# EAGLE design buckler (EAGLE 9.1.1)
AUTHOR: Branden Ghena; REV: B; TITLE: Berkeley Buckler

## Sheet 1 of 3: Headers
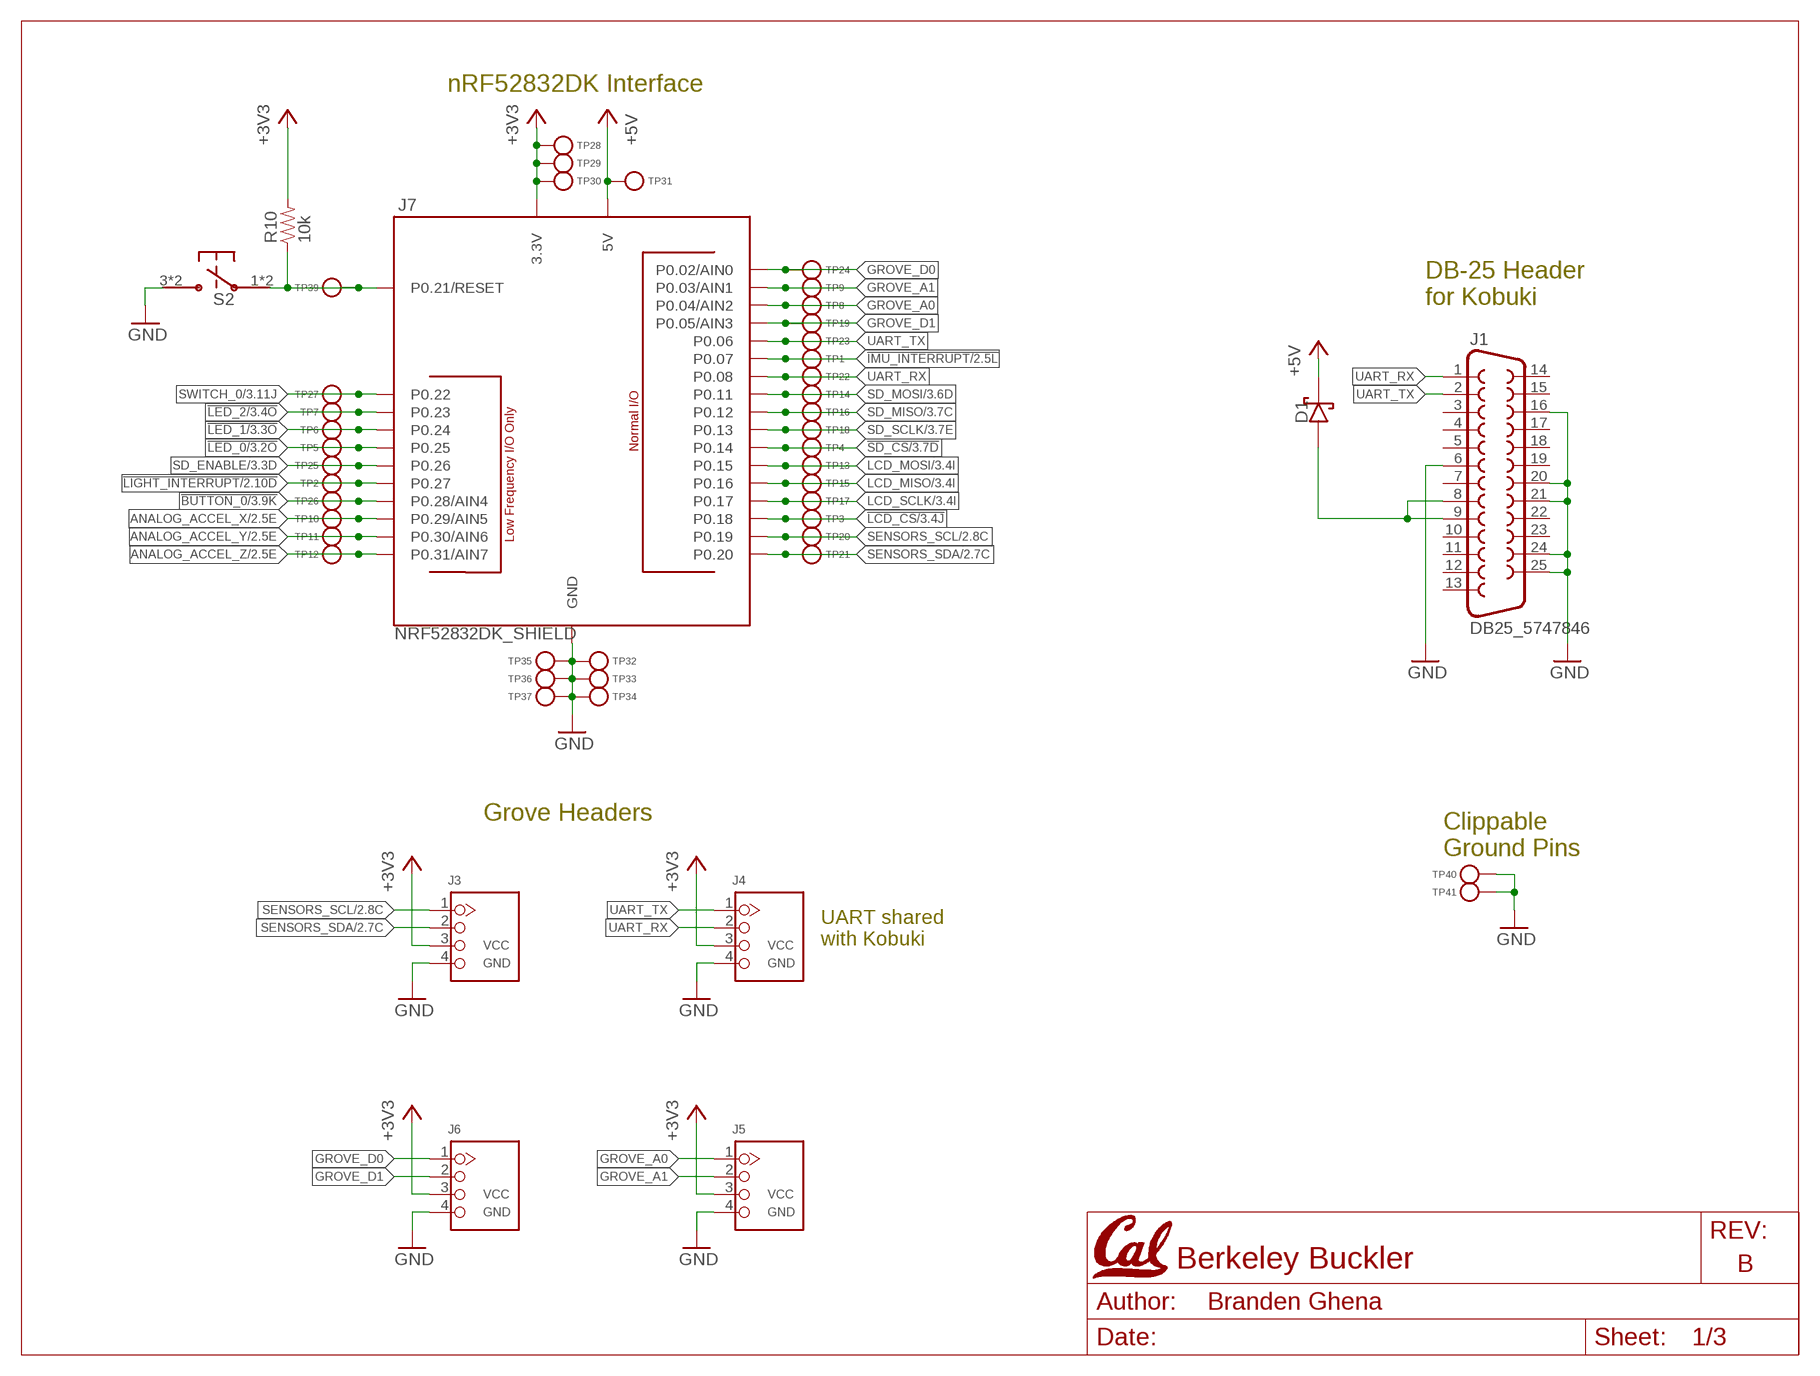
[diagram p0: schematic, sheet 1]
U$1 (LETTER_L_CAL): HEIGHT: 8.5in; WIDTH: 11in

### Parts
D1  DIODE_SCHOTTKYSOD323  [SOD323]
J1  DB25_5747846  [DB25_5747846]
J3  GROVE-CONNECTOR-DIP(4P-2.0)  [HW4-2.0]
J4  GROVE-CONNECTOR-DIP(4P-2.0)  [HW4-2.0]
J5  GROVE-CONNECTOR-DIP(4P-2.0)  [HW4-2.0]
J6  GROVE-CONNECTOR-DIP(4P-2.0)  [HW4-2.0]
J7  NRF52832DK_SHIELD  [NRF52832DK_SHIELD]
R10  10k  RESISTOR0402_RES  [0402_RES]
S2  PTS645SM43SMTR92  [PTS645]
TP1  TEST_POINT_0.040IN  [TESTPOINT_0.040IN]
TP2  TEST_POINT_0.040IN  [TESTPOINT_0.040IN]
TP3  TEST_POINT_0.040IN  [TESTPOINT_0.040IN]
TP4  TEST_POINT_0.040IN  [TESTPOINT_0.040IN]
TP5  TEST_POINT_0.040IN  [TESTPOINT_0.040IN]
TP6  TEST_POINT_0.040IN  [TESTPOINT_0.040IN]
TP7  TEST_POINT_0.040IN  [TESTPOINT_0.040IN]
TP8  TEST_POINT_0.040IN  [TESTPOINT_0.040IN]
TP9  TEST_POINT_0.040IN  [TESTPOINT_0.040IN]
TP10  TEST_POINT_0.040IN  [TESTPOINT_0.040IN]
TP11  TEST_POINT_0.040IN  [TESTPOINT_0.040IN]
TP12  TEST_POINT_0.040IN  [TESTPOINT_0.040IN]
TP13  TEST_POINT_0.040IN  [TESTPOINT_0.040IN]
TP14  TEST_POINT_0.040IN  [TESTPOINT_0.040IN]
TP15  TEST_POINT_0.040IN  [TESTPOINT_0.040IN]
TP16  TEST_POINT_0.040IN  [TESTPOINT_0.040IN]
TP17  TEST_POINT_0.040IN  [TESTPOINT_0.040IN]
TP18  TEST_POINT_0.040IN  [TESTPOINT_0.040IN]
TP19  TEST_POINT_0.040IN  [TESTPOINT_0.040IN]
TP20  TEST_POINT_0.040IN  [TESTPOINT_0.040IN]
TP21  TEST_POINT_0.040IN  [TESTPOINT_0.040IN]
TP22  TEST_POINT_0.040IN  [TESTPOINT_0.040IN]
TP23  TEST_POINT_0.040IN  [TESTPOINT_0.040IN]
TP24  TEST_POINT_0.040IN  [TESTPOINT_0.040IN]
TP25  TEST_POINT_0.040IN  [TESTPOINT_0.040IN]
TP26  TEST_POINT_0.040IN  [TESTPOINT_0.040IN]
TP27  TEST_POINT_0.040IN  [TESTPOINT_0.040IN]
TP28  TEST_POINT_0.040IN  [TESTPOINT_0.040IN]
TP29  TEST_POINT_0.040IN  [TESTPOINT_0.040IN]
TP30  TEST_POINT_0.040IN  [TESTPOINT_0.040IN]
TP31  TEST_POINT_0.040IN  [TESTPOINT_0.040IN]
TP32  TEST_POINT_0.040IN  [TESTPOINT_0.040IN]
TP33  TEST_POINT_0.040IN  [TESTPOINT_0.040IN]
TP34  TEST_POINT_0.040IN  [TESTPOINT_0.040IN]
TP35  TEST_POINT_0.040IN  [TESTPOINT_0.040IN]
TP36  TEST_POINT_0.040IN  [TESTPOINT_0.040IN]
TP37  TEST_POINT_0.040IN  [TESTPOINT_0.040IN]
TP39  TEST_POINT_0.040IN  [TESTPOINT_0.040IN]
TP40  TEST_POINT_0.078IN  [TESTPOINT_0.078IN]
TP41  TEST_POINT_0.078IN  [TESTPOINT_0.078IN]

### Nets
5V_IN: D1.P$2(ANODE) J1.8 J1.9
!BUTTON_0: J7.P0.28(P0.28/AIN4) TP26.TESTPOINT ; also sheet 3
!IMU_INTERRUPT: J7.P0.07 TP1.TESTPOINT ; also sheet 2
!LCD_CS: J7.P0.18 TP3.TESTPOINT ; also sheet 3
!LED_0: J7.P0.25 TP5.TESTPOINT ; also sheet 3
!LED_1: J7.P0.24 TP6.TESTPOINT ; also sheet 3
!LED_2: J7.P0.23 TP7.TESTPOINT ; also sheet 3
!LIGHT_INTERRUPT: J7.P0.27 TP2.TESTPOINT ; also sheet 2
!RESET: J7.P0.21(P0.21/RESET) R10.1 S2.1 S2.2 TP39.TESTPOINT
!SD_CS: J7.P0.14 TP4.TESTPOINT ; also sheet 3
+3V3: J3.3 J4.3 J5.3 J6.3 J7.3.3V@0(3.3V) J7.3.3V@1(3.3V) J7.3.3V@2(3.3V) R10.2 TP28.TESTPOINT TP29.TESTPOINT TP30.TESTPOINT ; also sheet 2,3
+5V: D1.P$1(CATHODE) J7.5V TP31.TESTPOINT
ANALOG_ACCEL_X: J7.P0.29(P0.29/AIN5) TP10.TESTPOINT ; also sheet 2
ANALOG_ACCEL_Y: J7.P0.30(P0.30/AIN6) TP11.TESTPOINT ; also sheet 2
ANALOG_ACCEL_Z: J7.P0.31(P0.31/AIN7) TP12.TESTPOINT ; also sheet 2
GND: J1.6 J1.16 J1.20 J1.21 J1.24 J1.25 J3.4 J4.4 J5.4 J6.4 J7.GND@0(GND) J7.GND@1(GND) J7.GND@2(GND) S2.3 S2.4 TP32.TESTPOINT TP33.TESTPOINT TP34.TESTPOINT TP35.TESTPOINT TP36.TESTPOINT TP37.TESTPOINT TP40.1(TESTPOINT) TP41.1(TESTPOINT) ; also sheet 2,3
GROVE_A0: J5.1 J7.P0.04(P0.04/AIN2) TP8.TESTPOINT
GROVE_A1: J5.2 J7.P0.03(P0.03/AIN1) TP9.TESTPOINT
GROVE_D0: J6.1 J7.P0.02(P0.02/AIN0) TP24.TESTPOINT
GROVE_D1: J6.2 J7.P0.05(P0.05/AIN3) TP19.TESTPOINT
LCD_MISO: J7.P0.16 TP15.TESTPOINT ; also sheet 3
LCD_MOSI: J7.P0.15 TP13.TESTPOINT ; also sheet 3
LCD_SCLK: J7.P0.17 TP17.TESTPOINT ; also sheet 3
SD_ENABLE: J7.P0.26 TP25.TESTPOINT ; also sheet 3
SD_MISO: J7.P0.12 TP16.TESTPOINT ; also sheet 3
SD_MOSI: J7.P0.11 TP14.TESTPOINT ; also sheet 3
SD_SCLK: J7.P0.13 TP18.TESTPOINT ; also sheet 3
SENSORS_SCL: J3.1 J7.P0.19 TP20.TESTPOINT ; also sheet 2
SENSORS_SDA: J3.2 J7.P0.20 TP21.TESTPOINT ; also sheet 2
SWITCH_0: J7.P0.22 TP27.TESTPOINT ; also sheet 3
UART_RX: J1.1 J4.2 J7.P0.08 TP22.TESTPOINT
UART_TX: J1.2 J4.1 J7.P0.06 TP23.TESTPOINT
Unconnected: J1.3 J1.4 J1.5 J1.7 J1.10 J1.11 J1.12 J1.13 J1.14 J1.15 J1.17 J1.18 J1.19 J1.22 J1.23

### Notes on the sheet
- nRF52832DK Interface
- DB-25 Header
  for Kobuki
- Grove Headers
- Clippable
  Ground Pins
- UART shared
  with Kobuki

## Sheet 2 of 3: Sensors
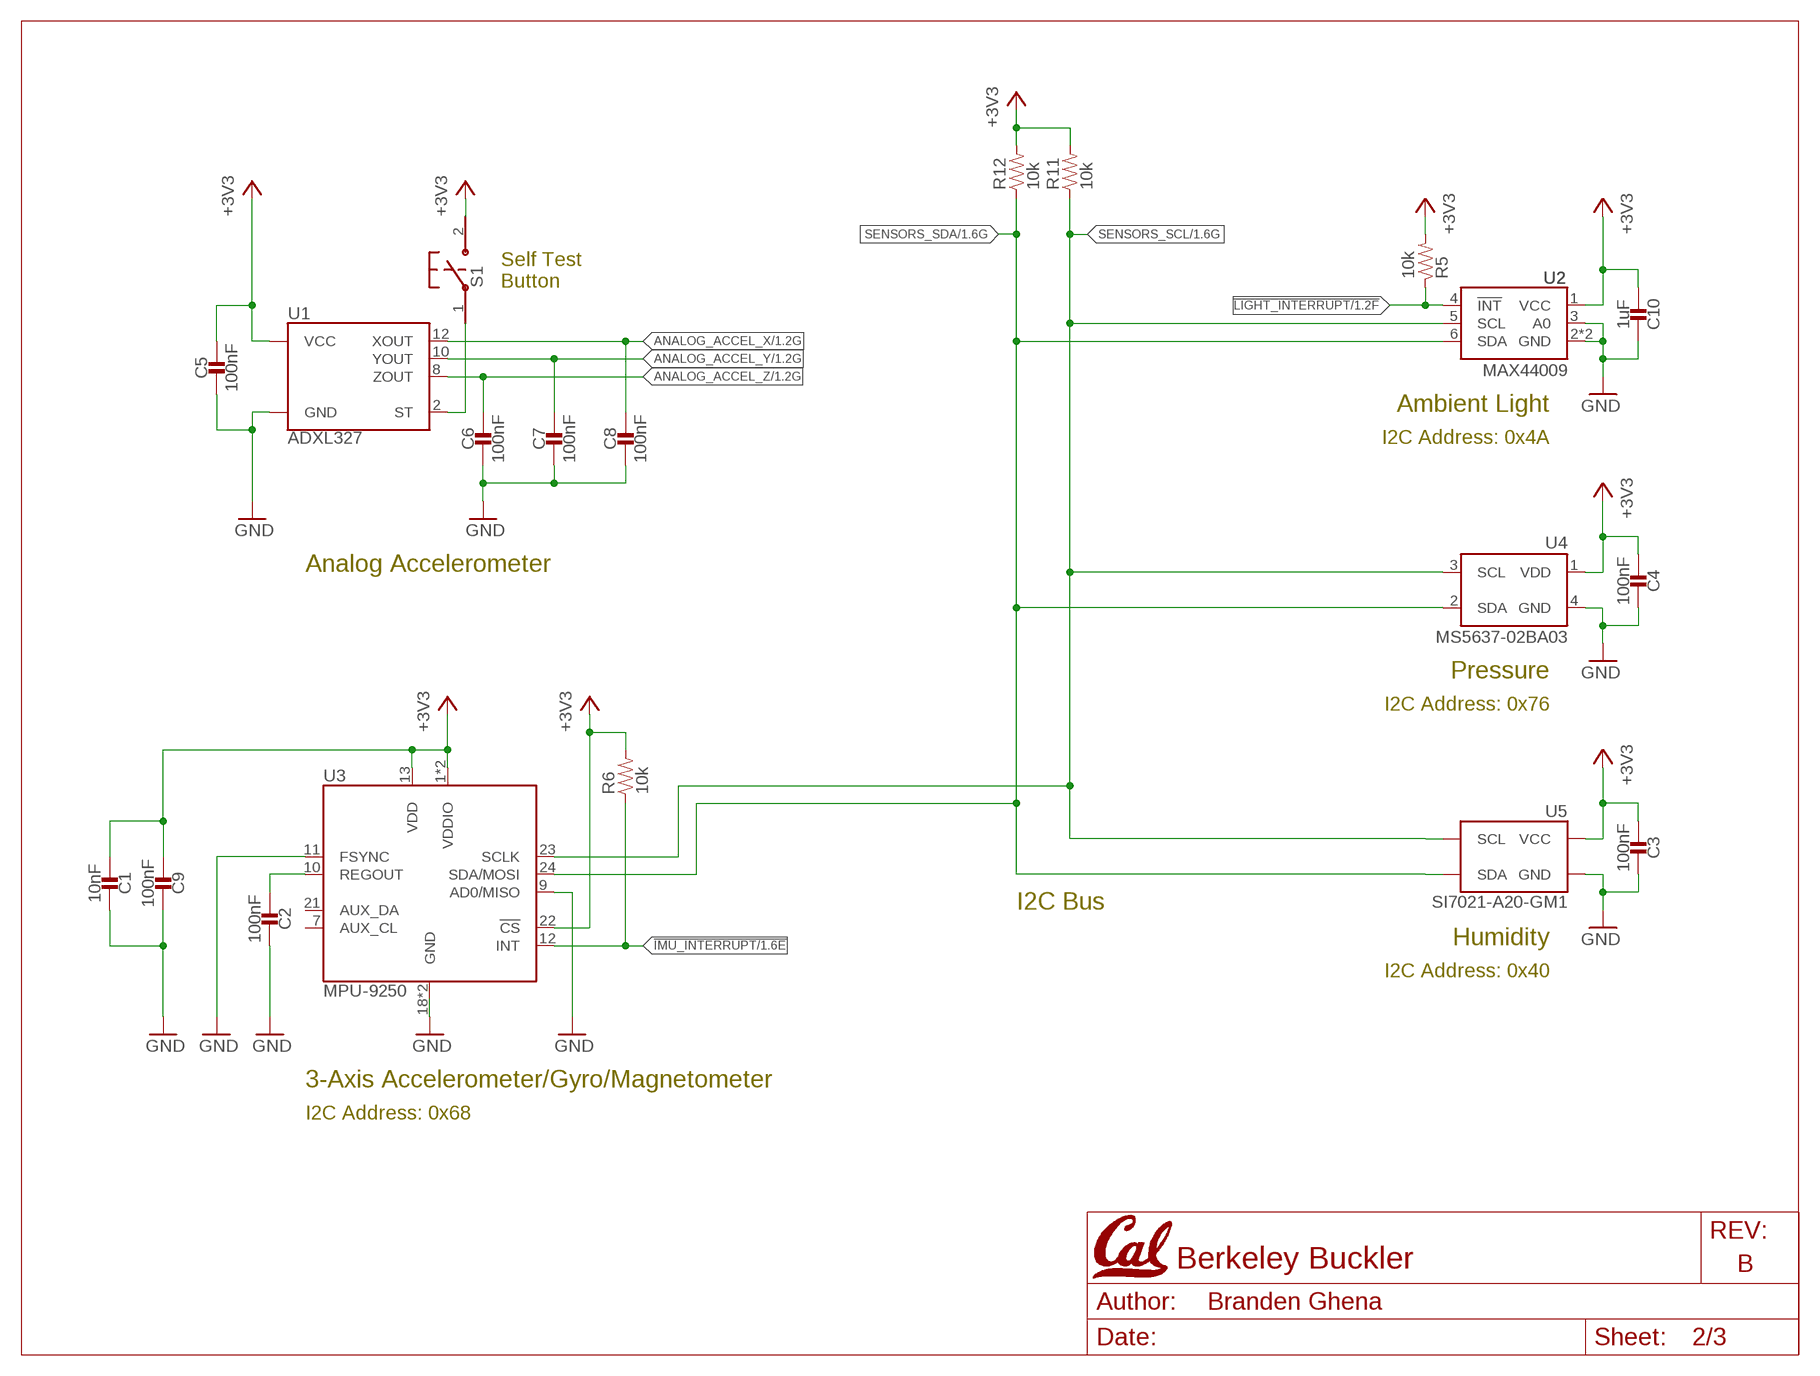
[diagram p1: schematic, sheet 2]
U$2 (LETTER_L_CAL): HEIGHT: 8.5in; WIDTH: 11in

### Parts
C1  10nF  CAPACITOR0402_CAP  [0402_CAP]
C2  100nF  CAPACITOR0402_CAP  [0402_CAP]
C3  100nF  CAPACITOR0402_CAP  [0402_CAP]
C4  100nF  CAPACITOR0402_CAP  [0402_CAP]
C5  100nF  CAPACITOR0402_CAP  [0402_CAP]
C6  100nF  CAPACITOR0402_CAP  [0402_CAP]
C7  100nF  CAPACITOR0402_CAP  [0402_CAP]
C8  100nF  CAPACITOR0402_CAP  [0402_CAP]
C9  100nF  CAPACITOR0402_CAP  [0402_CAP]
C10  1uF  CAPACITOR0402_CAP  [0402_CAP]
R5  10k  RESISTOR0402_RES  [0402_RES]
R6  10k  RESISTOR0402_RES  [0402_RES]
R11  10k  RESISTOR0402_RES  [0402_RES]
R12  10k  RESISTOR0402_RES  [0402_RES]
S1  B3U-1000P  [B3U-1000P]
U1  ADXL327  [LFCSP-16]
U2  MAX44009  [UDFN-6-EXPOSED]
U3  MPU-9250  [QFN-24/3MM]
U4  MS5637-02BA03  [4-SMD]
U5  SI7021-A20-GM1  [DFN-6/3MM]

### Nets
!IMU_INTERRUPT: R6.1 U3.12(INT) ; also sheet 1
!LIGHT_INTERRUPT: R5.1 U2.4(!INT) ; also sheet 1
+3V3: C1.1 C3.1 C4.1 C5.1 C9.1 C10.1 R5.2 R6.2 R11.2 R12.2 S1.2 U1.14(VCC) U1.15(VCC) U2.1(VCC) U3.1(VDDIO) U3.8(VDDIO) U3.13(VDD) U3.22(!CS) U4.1(VDD) U5.5(VCC) ; also sheet 1,3
ANALOG_ACCEL_X: C8.1 U1.12(XOUT) ; also sheet 1
ANALOG_ACCEL_Y: C7.1 U1.10(YOUT) ; also sheet 1
ANALOG_ACCEL_Z: C6.1 U1.8(ZOUT) ; also sheet 1
GND: C1.2 C2.2 C3.2 C4.2 C5.2 C6.2 C7.2 C8.2 C9.2 C10.2 U1.3(GND) U1.5(GND) U1.6(GND) U1.7(GND) U2.2(GND) U2.3(A0) U2.EP(GND) U3.9(AD0/MISO) U3.11(FSYNC) U3.18(GND) U3.20(GND) U4.4(GND) U5.2(GND) ; also sheet 1,3
N$7: S1.1 U1.2(ST)
N$19: C2.1 U3.10(REGOUT)
SENSORS_SCL: R11.1 U2.5(SCL) U3.23(SCLK) U4.3(SCL) U5.6(SCL) ; also sheet 1
SENSORS_SDA: R12.1 U2.6(SDA) U3.24(SDA/MOSI) U4.2(SDA) U5.1(SDA) ; also sheet 1
Unconnected: U3.7(AUX_CL) U3.21(AUX_DA)

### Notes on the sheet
- Self Test
  Button
- Ambient Light
- I2C Address: 0x4A
- Analog Accelerometer
- Pressure
- I2C Address: 0x76
- I2C Bus
- Humidity
- I2C Address: 0x40
- 3-Axis Accelerometer/Gyro/Magnetometer
- I2C Address: 0x68

## Sheet 3 of 3: Other Peripherals
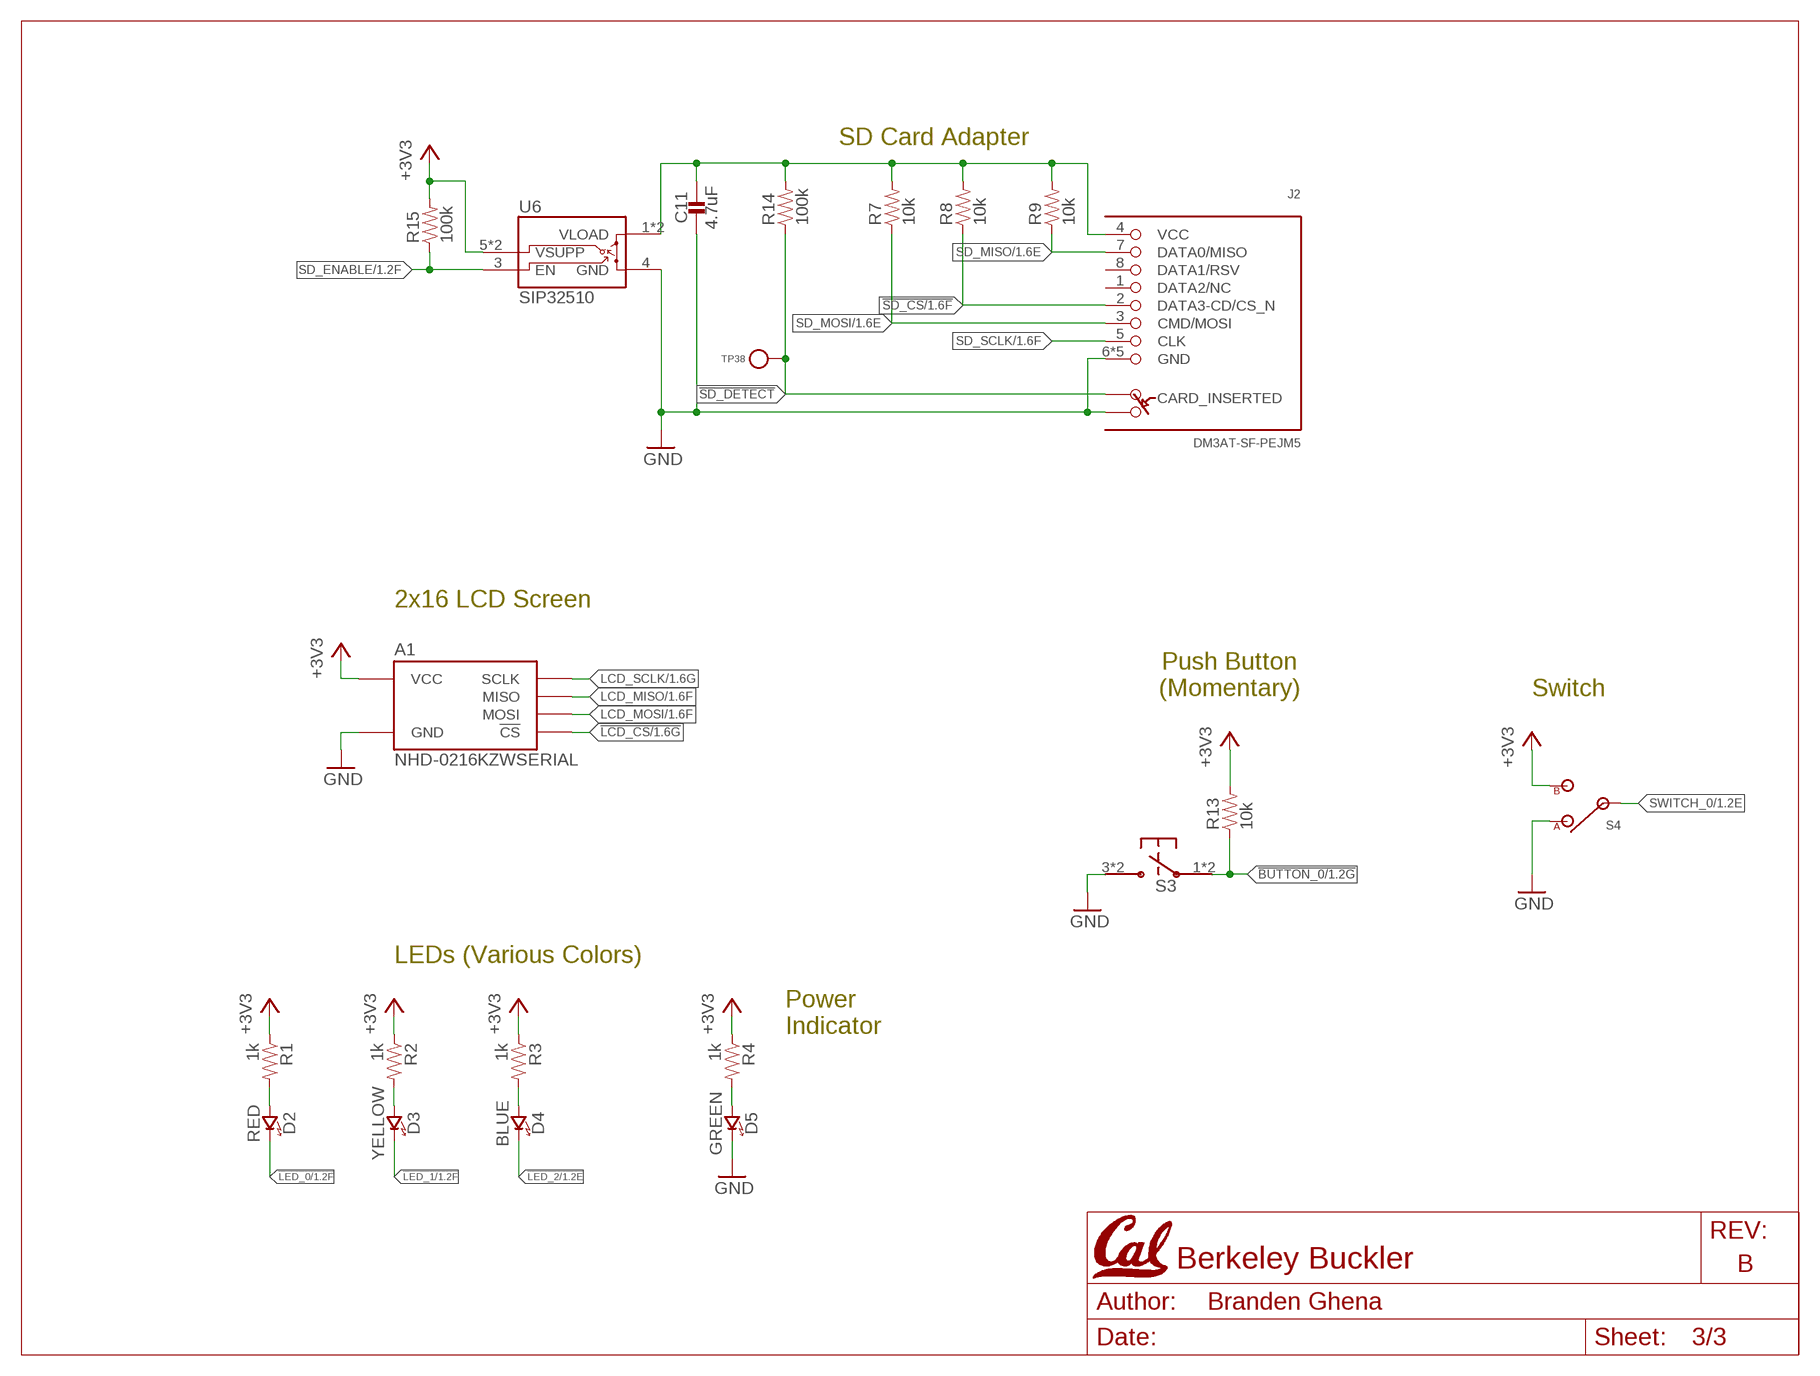
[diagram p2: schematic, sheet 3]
U$3 (LETTER_L_CAL): HEIGHT: 8.5in; WIDTH: 11in

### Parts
A1  NHD-0216KZWSERIAL  [NHD-0216KZW]
C11  4.7uF  CAPACITOR0402_CAP  [0402_CAP]
D2  RED  LED0603  [LED-0603]
D3  YELLOW  LED0603  [LED-0603]
D4  BLUE  LED0603  [LED-0603]
D5  GREEN  LED0603  [LED-0603]
J2  DM3AT-SF-PEJM5  [DM3AT-SF-PEJM5]
R1  1k  RESISTOR0402_RES  [0402_RES]
R2  1k  RESISTOR0402_RES  [0402_RES]
R3  1k  RESISTOR0402_RES  [0402_RES]
R4  1k  RESISTOR0402_RES  [0402_RES]
R7  10k  RESISTOR0402_RES  [0402_RES]
R8  10k  RESISTOR0402_RES  [0402_RES]
R9  10k  RESISTOR0402_RES  [0402_RES]
R13  10k  RESISTOR0402_RES  [0402_RES]
R14  100k  RESISTOR0402_RES  [0402_RES]
R15  100k  RESISTOR0402_RES  [0402_RES]
S3  PTS645SM43SMTR92  [PTS645]
S4  TE_SSA12/SPDT  [TE_SSA12/SPDT]
TP38  TEST_POINT_0.040IN  [TESTPOINT_0.040IN]
U6  SIP32510  [TSOT23-6]

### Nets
!BUTTON_0: R13.1 S3.1 S3.2 ; also sheet 1
!LCD_CS: A1.16(!CS) ; also sheet 1
!LED_0: D2.C(CATHODE) ; also sheet 1
!LED_1: D3.C(CATHODE) ; also sheet 1
!LED_2: D4.C(CATHODE) ; also sheet 1
!SD_CS: J2.2(DATA3-CD/CS_N) R8.1 ; also sheet 1
!SD_DETECT: J2.A R14.1 TP38.TESTPOINT
+3V3: A1.2(VCC) R1.1 R2.1 R3.1 R4.1 R13.2 R15.2 S4.2(B) U6.5(VSUPP) U6.6(VSUPP) ; also sheet 1,2
GND: A1.1(GND) C11.2 D5.C(CATHODE) J2.6(GND) J2.B J2.MOUNT0(GND) J2.MOUNT1(GND) J2.MOUNT2(GND) J2.MOUNT3(GND) S3.3 S3.4 S4.1(A) U6.4(GND) ; also sheet 1,2
LCD_MISO: A1.13(MISO) ; also sheet 1
LCD_MOSI: A1.14(MOSI) ; also sheet 1
LCD_SCLK: A1.12(SCLK) ; also sheet 1
N$3: D5.A(ANODE) R4.2
N$4: D4.A(ANODE) R3.2
N$5: D3.A(ANODE) R2.2
N$18: C11.1 J2.4(VCC) R7.2 R8.2 R9.2 R14.2 U6.1(VLOAD) U6.2(VLOAD)
N$25: D2.A(ANODE) R1.2
SD_ENABLE: R15.1 U6.3(EN) ; also sheet 1
SD_MISO: J2.7(DATA0/MISO) R9.1 ; also sheet 1
SD_MOSI: J2.3(CMD/MOSI) R7.1 ; also sheet 1
SD_SCLK: J2.5(CLK) ; also sheet 1
SWITCH_0: S4.IN ; also sheet 1
Unconnected: J2.1(DATA2/NC) J2.8(DATA1/RSV)

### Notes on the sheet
- SD Card Adapter
- 2x16 LCD Screen
- Push Button
  (Momentary)
- Switch
- LEDs (Various Colors)
- Power
  Indicator

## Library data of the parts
A1 = headers:NHD-0216KZW; DIGIKEY: NHD-0216KZW-AG5-ND,952-3305-ND; DIGIKEY1: NHD-0216KZW-AG5-ND; DIGIKEY2: 952-3305-ND; DIGIKEY3: 952-1862-ND
C1 = passives:CAPACITOR: SMD Capacitor; DESCRIPTION: CAP CER 10000PF 25V X7R 0402; DIGIKEY: 399-1279-1-ND; MANUFACTURER: KEMET; MPN: C0402C103J3RACTU
C2-C9 = passives:CAPACITOR: SMD Capacitor; DESCRIPTION: CAP CER 0.1UF 16V X7R 0402; DIGIKEY: 490-4759-1-ND; MANUFACTURER: Murata; MPN: GCM155R71C104KA55D
C10 = passives:CAPACITOR: SMD Capacitor; DESCRIPTION: CAP CER 1UF 10V X6S 0402; DIGIKEY: 1276-6805-1-ND; MANUFACTURER: Samsung Electro-Mechanics; MPN: CL05X105KP5NNNC
C11 = passives:CAPACITOR: SMD Capacitor; DESCRIPTION: CAP CER 4.7UF 10V X5R 0402; DIGIKEY: 1276-1480-1-ND; MANUFACTURER: Samsung Electro-Mechanics; MPN: CL05A475KP5NRNC
D1 = passives:DIODE_SCHOTTKY; DESCRIPTION: DIODE SCHOTTKY 30V 500MA SOD323; DIGIKEY: B0530WS-FDICT-ND; MANUFACTURER: Diodes Incorporated; MPN: B0530WS-7-F
D2 = leds:LED: LED; DESCRIPTION: LED RED CLEAR CHIP SMD; DIGIKEY: 160-1436-1-ND; MANUFACTURER: Lite-On Inc.; MPN: LTST-C190KRKT
D3 = leds:LED: LED; DESCRIPTION: LED YELLOW CLEAR CHIP SMD; DIGIKEY: 160-1437-1-ND; MANUFACTURER: Lite-On Inc.; MPN: LTST-C190KSKT
D4 = leds:LED: LED; DESCRIPTION: LED BLUE CLEAR SMD; DIGIKEY: 160-1837-1-ND; MANUFACTURER: Lite-On Inc.; MPN: LTST-C194TBKT
D5 = leds:LED: LED; DESCRIPTION: LED GREEN CLEAR CHIP SMD; DIGIKEY: 160-1435-1-ND; MANUFACTURER: Lite-On Inc.; MPN: LTST-C190KGKT
J1 = headers:DB25_5747846; DESCRIPTION: CONN D-SUB RCPT 25POS R/A SOLDER; DIGIKEY: A32126-ND; MANUFACTURER: TE Connectivity AMP Connectors; MPN: 5747846-4
J2 = connector:DM3AT-SF-PEJM5: CONN MICRO SD R/A PUSH-PUSH SMD; DESCRIPTION: CONN MICRO SD CARD PUSH-PUSH R/A; DIGIKEY: HR1964CT-ND; MANUFACTURER: Hirose Electric Co Ltd; MPN: DM3AT-SF-PEJM5
J3-J6 = headers:GROVE-CONNECTOR-DIP(4P-2.0): 320110033; DESCRIPTION: Grove - Universal 4 pin connector; MANUFACTURER: Seeed Studio; MOUSER: 713-110990030; MPN: 110990030; VALUE: 4P-2.0
J7 = headers:NRF52832DK_SHIELD: Shield for the PCA10040 nRF52832 Development Kit; DIGIKEY1: S1011EC-10-ND; DIGIKEY2: S1011EC-08-ND; DIGIKEY3: S1011EC-08-ND; DIGIKEY4: S1011EC-06-ND; DIGIKEY5: S1011EC-09-ND
R1-R4 = passives:RESISTOR: Resistor; DESCRIPTION: RES SMD 1K OHM 1% 1/16W 0402; DIGIKEY: RMCF0402FT1K00CT-ND; MANUFACTURER: Stackpole Electronics; MPN: RMCF0402FT1K00
R5-R13 = passives:RESISTOR: Resistor; DESCRIPTION: RES SMD 10K OHM 1% 1/16W 0402; DIGIKEY: 1276-3431-1-ND; MANUFACTURER: Samsung Electro-Mechanics; MPN: RC1005F103CS
R14 R15 = passives:RESISTOR: Resistor; DESCRIPTION: RES SMD 100K OHM 1% 1/5W 0402; DIGIKEY: 541-100KYCT-ND; MANUFACTURER: Vishay Dale; MPN: CRCW0402100KFKEDHP
S1 = switches:B3U: Switch; DESCRIPTION: SWITCH TACTILE SPST-NO 0.05A 12V; DIGIKEY: SW1020CT-ND; MANUFACTURER: Omron; MPN: B3U-1000P
S2 S3 = switches:PTS645SM43SMTR92: Tactile Switch SPST-NO Top Actuated Surface Mount; DESCRIPTION: SWITCH TACTILE SPST-NO 0.05A 12V; DIGIKEY: CKN9112CT-ND; MANUFACTURER: C&K; MPN: PTS645SM43SMTR92 LFS
S4 = switches:TE_SSA12/SPDT: SWITCH SLIDE SPDT 2POS SSA SER; DESCRIPTION: SWITCH SLIDE SPDT 100MA 30V; DIGIKEY: 450-1602-ND; MANUFACTURER: TE Connectivity ALCOSWITCH Switches; MPN: SSA12
TP1-TP39 = headers:TEST_POINT_0.040IN: 0.040in Test Point; DIGIKEY: 5001K-ND
TP40 TP41 = headers:TEST_POINT_0.078IN; DESCRIPTION: TERM TURRET SINGLE L=4.75MM TIN; DIGIKEY: 36-1520-2-ND; MANUFACTURER: Keystone Electronics; MPN: 1520-2
U1 = chips:ADXL327: ADXL327 3-Axis Analog Accelerometer; DESCRIPTION: ACCELEROMETER 2G ANALOG 16LFCSP; DIGIKEY: ADXL327BCPZ-ND; MANUFACTURER: Analog Devices Inc.; MPN: ADXL327BCPZ
U2 = chips:MAX44009: low power ambient light sensor; DESCRIPTION: SENSOR AMBIENT LIGHT 6UTDFN; DIGIKEY: MAX44009EDT+TCT-ND; MANUFACTURER: Maxim Integrated; MPN: MAX44009EDT+T
U3 = chips:MPU-9250: GYRO/ACCEL/COMPASS/9-AXIS; DESCRIPTION: IMU ACCEL/GYRO/MAG I2C/SPI 24QFN; DIGIKEY: 1428-1019-1-ND; MANUFACTURER: TDK InvenSense; MPN: MPU-9250
U4 = chips:MS5637-02BA03: low power pressure sensor; DESCRIPTION: SENSOR 17.4PSIA I2C 24B 4-QFN; DIGIKEY: 223-1199-1-ND; MANUFACTURER: TE CONNECTIVITY; MPN: MS563702BA03-50
U5 = chips:SI7021: IC TEMP SENSOR RH 2% DFN; DESCRIPTION: SENS HUMI/TEMP 3.6V I2C 3% 6DFN; DIGIKEY: 336-3141-ND; MANUFACTURER: Silicon Labs; MOUSER: 634-SI7021-A20-GM1; MPN: SI7021-A20-GM1
U6 = chips:SIP32510: Load switch, slew rate controlled. By Vishay; DESCRIPTION: IC LOAD SWITCH SOT23-6; DIGIKEY: SIP32510DT-T1-GE3CT-ND; MANUFACTURER: Vishay; MPN: SIP32510DT-T1-GE3

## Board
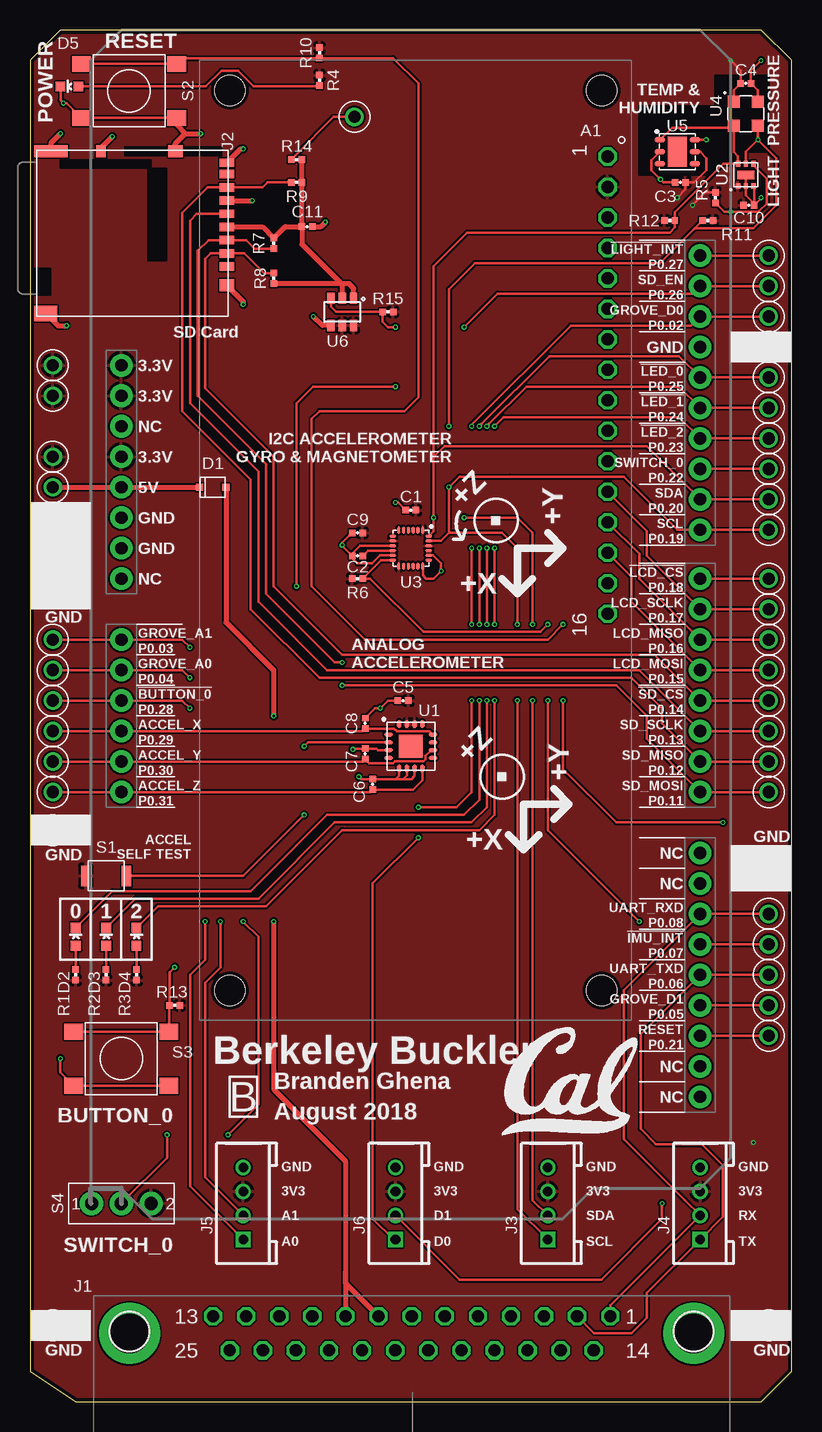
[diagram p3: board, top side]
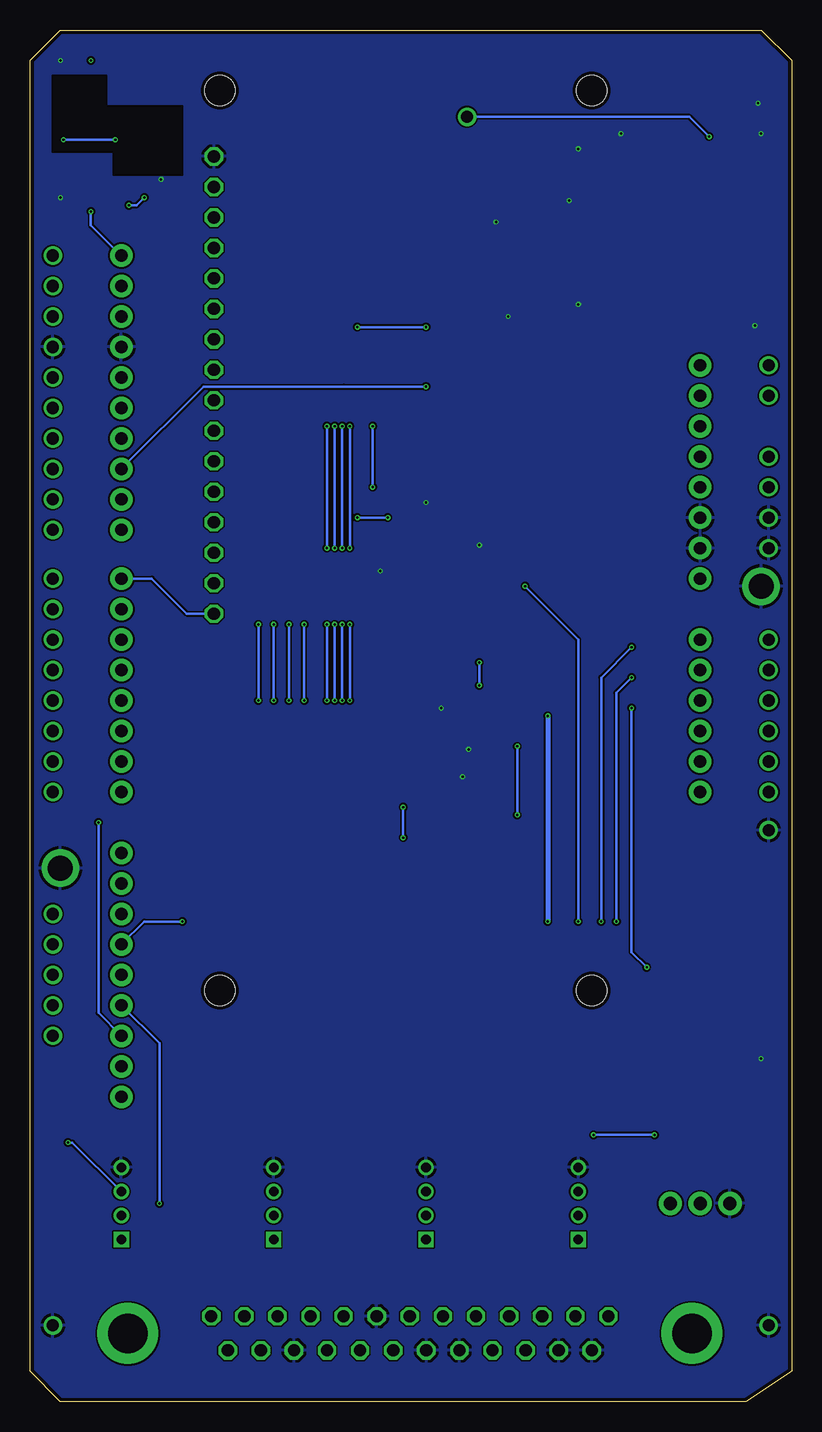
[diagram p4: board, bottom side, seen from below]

Size 63.5 x 114.3 mm. Coordinates in mm from the lower left corner, seen from the top.
Outline: 60.96,114.3 2.54,114.3 0,111.76 0,2.54 3.81,0 8.89,0 43.18,0 46.99,0 55.88,0 58.42,0 60.96,0 63.5,2.54 63.5,111.76 60.96,114.3
Copper layers (1*16): Top 0.0178mm / dielectric 59mil / Bottom 0.0178mm
Design rules "quickturn_co_kr_1oz": minimum track width 4mil, minimum drill 0.200659375mm, track to track 6mil, track to pad 6mil, pad to pad 6mil, via to via 6mil, smd to smd 6mil, copper to edge 12mil, drill to drill 12mil, minimum pad ring 8mil, minimum via ring 4mil, stop-mask expansion 3mil, vias tented up to drill 50mil, thermal gap 10mil

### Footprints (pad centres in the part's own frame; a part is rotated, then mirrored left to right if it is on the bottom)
NHD-0216KZW = drill 1.016 octagon: 1 8,-2; 2 10.54,-2; 3 13.08,-2; 4 15.62,-2; 5 18.16,-2; 6 20.7,-2; 7 23.24,-2; 8 25.78,-2; 9 28.32,-2; 10 30.86,-2; 11 33.4,-2; 12 35.94,-2; 13 38.48,-2; 14 41.02,-2; 15 43.56,-2; 16 46.1,-2 | hole 2.5: 2.5,-2.5; 2.5,-33.5; 77.5,-33.5; 77.5,-2.5
0402_CAP = smd 0.536 x 0.546: 1 -0.433,0; 2 0.433,0
SOD323 = smd 0.6 x 0.6: P$1 -1.1,0; P$2 1.1,0
LED-0603 = smd 0.8 x 0.8: A 0,-0.75; C 0,0.75
DB25_5747846 = drill 1.016 octagon: 1 0,0; 2 2.76,0; 3 5.52,0; 4 8.28,0; 5 11.041,0; 6 13.801,0; 7 16.561,0; 8 19.321,0; 9 22.081,0; 10 24.841,0; 11 27.601,0; 12 30.362,0; 13 33.122,0; 14 1.379,2.845; 15 4.139,2.845; 16 6.898,2.845; 17 9.657,2.845; 18 12.417,2.845; 19 15.176,2.845; 20 17.935,2.845; 21 20.695,2.845; 22 23.454,2.845; 23 26.213,2.845; 24 28.973,2.845; 25 31.732,2.845 | drill 3.302 pad 5.08: G1 -6.96,1.422; G2 40.081,1.422
DM3AT-SF-PEJM5 = smd 0.7 x 1.2: 1 3.2,-0.1; 2 2.1,-0.1; 3 1,-0.1; 4 -0.1,-0.1; 5 -1.2,-0.1; 6 -2.3,-0.1; 7 -3.4,-0.1; 8 -4.5,-0.1; B -5.45,-0.1 | smd 1 x 0.8: A -6.4,-10.6 | smd 1 x 1.2: MOUNT0 4.75,-0.1; MOUNT1 -6.4,-4.4 | smd 1 x 2.8: MOUNT2 -6.4,-14.75 | smd 1.3 x 1.9: MOUNT3 7.1,-15.2
HW4-2.0 = drill 0.8 pad 1.27 square: 1 -3,0 | drill 0.8 pad 1.27: 2 -1,0; 3 1,0; 4 3,0
NRF52832DK_SHIELD = drill 1.016 pad 1.88: 3.3V@0 0,-7.62; 3.3V@1 0,-2.54; 3.3V@2 0,0; 5V 0,-10.16; !RESET 0,-5.08; GND@0 0,-12.7; GND@1 0,-15.24; GND@2 48.26,1.524; NC@0 0,-17.78; NC@1 48.26,-58.42; NC@2 48.26,-60.96; P0.02 48.26,4.064; P0.03 0,-22.86; P0.04 0,-25.4; P0.05 48.26,-53.34; P0.06 48.26,-50.8; P0.07 48.26,-48.26; P0.08 48.26,-45.72; P0.09 48.26,-43.18; P0.10 48.26,-40.64; P0.11 48.26,-35.56; P0.12 48.26,-33.02; P0.13 48.26,-30.48; P0.14 48.26,-27.94; P0.15 48.26,-25.4; P0.16 48.26,-22.86; P0.17 48.26,-20.32; P0.18 48.26,-17.78; P0.19 48.26,-13.716; P0.20 48.26,-11.176; P0.21 48.26,-55.88; P0.22 48.26,-8.636; P0.23 48.26,-6.096; P0.24 48.26,-3.556; P0.25 48.26,-1.016; P0.26 48.26,6.604; P0.27 48.26,9.144; P0.28 0,-27.94; P0.29 0,-30.48; P0.30 0,-33.02; P0.31 0,-35.56
0402_RES = smd 0.536 x 0.546: 1 -0.433,0; 2 0.433,0
B3U-1000P = smd 0.8 x 1.7: 1 -1.7,0; 2 1.7,0
PTS645 = smd 1.55 x 1.3: 1 -3.975,2.25; 2 3.975,2.25; 3 3.975,-2.25; 4 -3.975,-2.25
TE_SSA12/SPDT = drill 1.092 pad 1.93: 1 -2.489,0; 2 2.489,0; IN 0,0
TESTPOINT_0.040IN = drill 1.016: TESTPOINT 0,0
TESTPOINT_0.078IN = drill 2.083: 1 0,0
LFCSP-16 = smd 0.7 x 0.35: 1 -1.85,0.975; 2 -1.85,0.325; 3 -1.85,-0.325; 4 -1.85,-0.975; 9 1.85,-0.975; 10 1.85,-0.325; 11 1.85,0.325; 12 1.85,0.975 | smd 0.35 x 0.7: 5 -0.975,-1.85; 6 -0.325,-1.85; 7 0.325,-1.85; 8 0.975,-1.85; 13 0.975,1.85; 14 0.325,1.85; 15 -0.325,1.85; 16 -0.975,1.85 | smd 1.95 x 1.95: PAD 0,0
UDFN-6-EXPOSED = smd 0.48 x 0.36: 1 -0.925,0.65; 2 -0.925,0; 3 -0.925,-0.65; 4 0.925,-0.65; 5 0.925,0; 6 0.925,0.65 | smd 0.71 x 1.4: EP 0,0
QFN-24/3MM = smd 0.6 x 0.23: 1 -1.5,1; 2 -1.5,0.6; 3 -1.5,0.2; 4 -1.5,-0.2; 5 -1.5,-0.6; 6 -1.5,-1; 13 1.5,-1; 14 1.5,-0.6; 15 1.5,-0.2; 16 1.5,0.2; 17 1.5,0.6; 18 1.5,1 | smd 0.23 x 0.6: 7 -1,-1.5; 8 -0.6,-1.5; 9 -0.2,-1.5; 10 0.2,-1.5; 11 0.6,-1.5; 12 1,-1.5; 19 1,1.5; 20 0.6,1.5; 21 0.2,1.5; 22 -0.2,1.5; 23 -0.6,1.5; 24 -1,1.5
4-SMD = smd 1 x 1: 1 -1,1; 2 -1,-1; 3 1,-1; 4 1,1
DFN-6/3MM = smd 0.85 x 0.45: 1 -1.45,1; 2 -1.45,0; 3 -1.45,-1; 4 1.45,-1; 5 1.45,0; 6 1.45,1 | smd 1.6 x 2.5: P$1 0,0
TSOT23-6 = smd 0.6 x 0.927: 1 -0.95,-1.126; 2 0,-1.126; 3 0.95,-1.126; 4 0.95,1.126; 5 0,1.126; 6 -0.95,1.126

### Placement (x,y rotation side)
A1  50.16,111.76 270 top
C1  31.75,74.29 180 top
C2  27.3,70.48 180 top
C3  54.23,101.6 180 top
C4  59.69,109.85 0 top
C5  31.11,58.42 180 top
C6  28.57,51.44 90 top
C7  27.94,53.98 90 top
C8  27.94,56.52 90 top
C9  27.3,72.39 180 top
C10  59.94,99.69 0 top
C11  23.11,97.92 0 top
D1  15.24,76.2 0 top
D2  3.81,38.73 0 top
D3  6.35,38.73 0 top
D4  8.89,38.73 0 top
D5  3.3,109.6 90 top
J1  48.39,7.11 180 top
J2  16.51,97.79 270 top
J3  43.18,16.51 90 top
J4  55.88,16.51 90 top
J5  17.78,16.51 90 top
J6  30.48,16.51 90 top
J7  7.62,86.36 0 top
R1  3.81,35.56 90 top
R2  6.35,35.56 90 top
R3  8.89,35.56 90 top
R4  24.13,110.11 270 top
R5  57.15,100.33 90 top
R6  27.3,68.58 180 top
R7  20.32,96.52 90 top
R8  20.32,93.6 270 top
R9  22.23,101.6 0 top
R10  24.13,112.39 90 top
R11  56.52,98.42 0 top
R12  53.34,98.42 180 top
R13  12.06,33.02 0 top
R14  22.23,103.5 0 top
R15  29.84,90.8 0 top
S1  6.35,43.82 180 top
S2  8.26,109.22 0 top
S3  7.62,28.58 0 top
S4  7.62,16.51 0 top
TP1  61.59,38.1 0 top
TP2  61.59,95.5 0 top
TP3  61.59,68.58 0 top
TP4  61.59,58.42 0 top
TP5  61.59,85.34 0 top
TP6  61.59,82.8 0 top
TP7  61.59,80.26 0 top
TP8  1.91,60.96 0 top
TP9  1.91,63.5 0 top
TP10  1.91,55.88 0 top
TP11  1.91,53.34 0 top
TP12  1.91,50.8 0 top
TP13  61.59,60.96 0 top
TP14  61.59,50.8 0 top
TP15  61.59,63.5 0 top
TP16  61.59,53.34 0 top
TP17  61.59,66.04 0 top
TP18  61.59,55.88 0 top
TP19  61.59,33.02 0 top
TP20  61.59,72.64 0 top
TP21  61.59,75.18 0 top
TP22  61.59,40.64 0 top
TP23  61.59,35.56 0 top
TP24  61.59,90.42 0 top
TP25  61.59,92.96 0 top
TP26  1.91,58.42 0 top
TP27  61.59,77.72 0 top
TP28  1.91,86.36 0 top
TP29  1.91,83.82 0 top
TP30  1.91,78.74 0 top
TP31  1.91,76.2 0 top
TP32  1.91,73.66 0 top
TP33  1.91,71.12 0 top
TP34  61.59,87.88 0 top
TP35  61.59,6.35 0 top
TP36  1.91,6.35 0 top
TP37  1.91,47.62 0 top
TP38  27.05,107.06 0 top
TP39  61.59,30.48 0 top
TP40  60.96,44.45 0 top
TP41  2.54,67.94 0 top
U1  31.75,54.61 0 top
U2  59.69,102.23 90 top
U3  31.75,71.12 270 top
U4  59.69,107.31 0 top
U5  53.98,104.14 0 top
U6  26.04,90.8 180 top
U$5  [UCB_CAL_350MIL]  39.37,22.23 0 top

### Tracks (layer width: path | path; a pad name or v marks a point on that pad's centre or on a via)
5V_IN  (via drill 0.2)
  Top 0.406: D1.P$2 16.34,64.94 20.32,60.96 v20.32,57.15 | v20.32,40.01 20.32,26.03 26.31,20.05 26.31,10.79 | 26.31,10.79 J1.9 | J1.8 26.31,9.87 26.31,10.79
  Bottom 0.406: v20.32,57.15 v20.32,40.01
!BUTTON_0  (via drill 0.2)
  Top 0.203: TP26.TESTPOINT J7.P0.28 12.7,58.42 v13.34,57.79 | S3.1 S3.2 11.6,32.98 R13.1 11.63,35.76 v12.06,36.2
  Bottom 0.203: v13.34,57.79 13.34,37.46 v12.06,36.2
!IMU_INTERRUPT  (via drill 0.2)
  Top 0.203: J7.P0.07 TP1.TESTPOINT | U3.12 29.28,70.12 R6.1 28.37,68.58 32.82,64.13 42.55,64.13 v43.18,64.77 | v50.8,40.01 43.18,47.62 v43.18,58.42
  Bottom 0.203: J7.P0.07 53.98,40.01 v50.8,40.01 | v43.18,58.42 v43.18,64.77
!LCD_CS
  Top 0.203: TP3.TESTPOINT J7.P0.18
  Bottom 0.203: J7.P0.18 53.34,68.58 50.42,65.66 A1.16
!LED_0  (via drill 0.2)
  Top 0.203: TP5.TESTPOINT J7.P0.25 54.1,87.12 43.3,87.12 37.64,81.47 37.64,81.46 v37.47,81.28 | D2.C 6.87,42.55 18.41,42.55 24.77,48.9 36.2,48.9 37.47,50.16 v37.47,58.42 | v37.47,64.77 v37.47,71.12
  Bottom 0.203: v37.47,58.42 v37.47,64.77 | v37.47,71.12 v37.47,81.28
!LED_1  (via drill 0.2)
  Top 0.203: TP6.TESTPOINT J7.P0.24 54.1,84.58 41.39,84.58 38.28,81.47 38.28,81.46 v38.1,81.28 | D3.C 8.78,41.91 19.05,41.91 25.4,48.26 36.83,48.26 38.1,49.53 v38.1,58.42 | v38.1,64.77 v38.1,71.12
  Bottom 0.203: v38.1,58.42 v38.1,64.77 | v38.1,71.12 v38.1,81.28
!LED_2  (via drill 0.2)
  Top 0.203: TP7.TESTPOINT J7.P0.23 54.1,82.04 39.5,82.04 v38.73,81.28 | D4.C 10.68,41.27 19.68,41.27 26.04,47.62 37.47,47.62 38.73,48.9 v38.73,58.42 | v38.73,64.77 v38.73,71.12
  Bottom 0.203: v38.73,58.42 v38.73,64.77 | v38.73,71.12 v38.73,81.28
!LIGHT_INTERRUPT  (via drill 0.2)
  Top 0.203: J7.P0.27 TP2.TESTPOINT | U2.4 60.34,103 61.42,101.92 61.42,99.83 60.8,99.22 | 60.8,99.22 60.75,99.17 | 60.8,99.22 60.75,99.17 | 60.75,99.17 v58.42,99.17 57.88,99.17 R5.1
  Bottom 0.203: v58.42,99.17 58.42,98.04 J7.P0.27
!RESET  (via drill 0.2)
  Top 0.203: J7.P0.21 TP39.TESTPOINT | S2.1 S2.2 12.72,111.96 R10.1 30.28,111.96 32.38,109.85 32.38,83.69 31.24,82.55 24.13,82.55 23.5,81.91 23.5,67.94 27.94,63.5 43.18,63.5 v44.45,64.77 | v44.45,58.42 44.45,52.7 48.9,48.26 v57.78,48.26
  Bottom 0.203: v44.45,64.77 v44.45,58.42 | J7.P0.21 57.78,32.38 v57.78,48.26
!SD_CS
  Top 0.203: TP4.TESTPOINT J7.P0.14 52.07,62.23 26.04,62.23 20.32,67.94 20.32,78.74 14.61,84.45 14.61,95.25 15.04,95.69 J2.2 17.85,95.69 19.51,94.03 R8.1
!SD_DETECT  (via drill 0.2)
  Top 0.203: J2.A 5.91,104.46 | R14.1 22.14,103.85 22.14,103.88 25.31,107.06 TP38.TESTPOINT
  Top 0.406: 5.91,104.46 v6.86,105.41
  Bottom 0.203: v6.86,105.41 8.51,107.06 TP38.TESTPOINT
+3V3  (via drill 0.2)
  Top 0.203: U4.1 58.69,109.29 C4.1 59.26,110.92 | U5.5 55.88,104.14 56.39,103.63 56.39,102.62 55.37,101.6 C3.1 54.66,101.02 v53.98,100.33 | R5.2 56.31,100.76 v55.24,99.69 | 59.26,110.92 | 59.26,110.92 v58.42,111.76
  Bottom 0.203: v55.24,99.69 54.61,99.69 v53.98,100.33 | J4.3 59.96,21.59 v60.33,21.59
  pour Top: -4.45,113.66 1.27,119.38 68.58,119.38 74.93,113.03 74.93,1.9 70.48,-2.54 -4.45,-2.54 -6.99,0 -6.99,1.27 -6.99,111.12
+5V
  Top 0.406: TP31.TESTPOINT J7.5V D1.P$1
ANALOG_ACCEL_X
  Top 0.203: TP10.TESTPOINT J7.P0.29 27.74,55.88 C8.1 30.37,56.08 30.6,55.86 33.33,55.86 U1.12
ANALOG_ACCEL_Y
  Top 0.203: TP11.TESTPOINT J7.P0.30 27.74,53.34 C7.1 28.28,53.21 30.25,53.21 30.43,53.38 32.83,53.38 33,53.55 33,53.81 33.47,54.29 U1.10
ANALOG_ACCEL_Z
  Top 0.203: TP12.TESTPOINT J7.P0.31 28.37,50.8 C6.1 31.95,51 32.73,51.77 U1.8
GND  (via drill 0.2)
  Top 0.203: S2.3 S2.4 3.05,108.2 v2.79,108.2 2.55,108.45 D5.C | S3.3 S3.4 2.54,27.43 v2.54,28.58 | U5.2 51.82,103.43 51.82,102.62 v52.58,101.85 52.83,101.6 C3.2 | U4.4 60.69,109.29 C4.2 60.12,110.92 v60.96,111.76 | U2.3 60.38,101.27 60.38,99.82 | 60.38,99.82 C10.2 60.96,100.28 v60.96,100.33 | U2.EP U2.2 59.69,100.51 60.38,99.82 | U1.7 32.08,52.14 31.8,51.87 31.11,51.87 | 30.48,51.87 31.11,51.87 | U1.6 31.43,52.18 31.11,51.87 | U1.5 30.77,52.16 30.48,51.87 | v27.43,52.07 27.63,51.87 C6.2 30.48,51.87 | C8.2 28.78,57.79 v29.21,57.79 29.84,58.42 C5.2 | U1.3 29.03,54.29 28.9,54.41 C7.2 26.98,54.41 v26.92,54.36 | C9.2 26.04,71.55 v26.04,71.37 26.04,71.32 26.77,70.59 | 26.77,70.59 C2.2 26.87,70.28 27.3,69.85 28.5,69.85 29.18,70.52 U3.11 | U3.9 27.5,71.32 26.77,70.59 | C1.2 30.68,74.93 v30.48,74.93 | U3.18 32.75,68.85 33.02,68.58 33.66,68.58 v34.29,69.22 34.29,69.85 33.62,70.52 U3.20
  Top 0.406: J2.MOUNT2 1.76,104.88 v2.54,105.66 | J2.MOUNT3 2.34,89.66 v3.05,89.66 | J2.B 17.56,104.39 v17.78,104.39 | J2.6 16.42,100.08 v18.54,100.08 | J2.MOUNT0 17.78,91.67 v17.78,91.44 | U6.4 24.37,89.68 v23.62,90.42 | C11.2 24.26,97.92 v24.64,98.3 | J2.MOUNT1 12.11,104.82 12.95,105.66 | 12.95,105.66 v14.22,105.66 | S2.3 12.23,106.39 12.95,105.66
  pour Bottom: -5.08,116.84 63.5,116.84 67.31,113.03 67.31,3.81 62.23,-1.27 0,-1.27 -7.62,6.35 -7.62,114.3
GROVE_A0  (via drill 0.2)
  Top 0.203: TP8.TESTPOINT J7.P0.04 12.7,60.96 v13.34,60.33 | v14.61,40.01 14.61,36.83 13.34,35.56 13.34,17.95 J5.1
  Bottom 0.203: v13.34,60.33 14.61,59.05 v14.61,40.01
GROVE_A1  (via drill 0.2)
  Top 0.203: TP9.TESTPOINT J7.P0.03 12.7,63.5 v13.34,62.87 | v15.88,40.01 15.88,36.2 14.61,34.92 14.61,18.69 J5.2
  Bottom 0.203: v13.34,62.87 15.88,60.33 v15.88,40.01
GROVE_D0  (via drill 0.2)
  Top 0.203: TP24.TESTPOINT J7.P0.02 55.12,89.66 45.09,89.66 36.83,81.41 v36.83,81.28 | v36.83,71.12 v36.83,64.77 | v36.83,58.42 36.83,50.8 35.56,49.53 v32.38,49.53 | v32.38,46.99 28.57,43.18 28.57,15.24 30.3,13.51 J6.1
  Bottom 0.203: v36.83,81.28 v36.83,71.12 | v36.83,64.77 v36.83,58.42 | v32.38,49.53 v32.38,46.99
GROVE_D1  (via drill 0.2)
  Top 0.203: TP19.TESTPOINT J7.P0.05 | J6.2 35.83,10.16 47.62,10.16 52.7,15.24 v52.7,16.51
  Bottom 0.203: v52.7,16.51 52.7,29.84 J7.P0.05
LCD_MISO
  Top 0.203: TP15.TESTPOINT J7.P0.16 50.8,68.58 50.8,70.64 A1.13
LCD_MOSI
  Top 0.203: TP13.TESTPOINT J7.P0.15 50.16,66.67 50.16,68.74 A1.14
LCD_SCLK
  Top 0.203: TP17.TESTPOINT J7.P0.17 51.44,70.48 51.44,72.55 A1.12
N$3
  Top 0.203: R4.2 24.05,109.6 18.67,109.6 17.35,110.92 15.98,110.92 14.66,109.6 D5.A
N$4
  Top 0.203: D4.A R3.2
N$5
  Top 0.203: D3.A R2.2
N$7  (via drill 0.2)
  Top 0.203: S1.1 17.78,43.82 v22.86,48.9 | v22.86,54.61 23.18,54.94 U1.2
  Bottom 0.203: v22.86,48.9 v22.86,54.61
N$18
  Top 0.406: R14.2 R9.2 22.66,97.94 C11.1 | J2.4 19.38,97.89 R7.2 21.28,97.92 C11.1 | C11.1 22.68,96.44 25.96,93.17 | 25.96,93.17 R8.2 | 25.96,93.17 26.04,93.09 U6.2 | U6.1 26.98,92.78 26.59,93.17 25.96,93.17
N$19
  Top 0.203: C2.1 28.17,70.92 U3.10
N$25
  Top 0.203: D2.A R1.2
N$50
  cutout Top: 56.52,102.23 50.8,102.23 50.8,107.95 55.88,107.95 57.15,107.95 57.15,110.49 61.59,110.49 61.59,104.14 56.52,104.14
N$51
  cutout Bottom: 56.52,102.23 50.8,102.23 50.8,107.95 57.15,107.95 57.15,110.49 61.59,110.49 61.59,104.14 56.52,104.14
SD_ENABLE  (via drill 0.2)
  Top 0.203: TP25.TESTPOINT J7.P0.26 55.24,92.33 38.99,92.33 v36.2,89.53 | U6.3 25.09,91.25 25.53,90.8 R15.1 29.41,89.97 29.84,89.53 v30.48,89.53
  Bottom 0.203: v30.48,89.53 v36.2,89.53
SD_MISO
  Top 0.203: TP16.TESTPOINT J7.P0.12 52.7,56.52 52.7,57.79 50.16,60.33 24.13,60.33 18.41,66.04 18.41,76.83 12.7,82.55 12.7,99.06 14.83,101.19 J2.7 19.4,101.19 19.81,101.6 R9.1
SD_MOSI  (via drill 0.2)
  Top 0.203: TP14.TESTPOINT J7.P0.11 51.44,55.25 51.44,57.15 48.9,59.69 v26.04,59.69 | R7.1 18.72,96.09 18.03,96.77 16.43,96.77 J2.3 14.88,96.79 13.97,95.88 13.97,83.82 19.68,78.1 19.68,67.31 25.4,61.59 v26.04,61.59
  Bottom 0.203: v26.04,61.59 v26.04,59.69
SD_SCLK
  Top 0.203: TP18.TESTPOINT J7.P0.13 53.98,57.79 50.8,60.96 24.77,60.96 19.05,66.67 19.05,77.47 13.34,83.18 13.34,98.42 13.9,98.99 J2.5
SENSORS_SCL  (via drill 0.2)
  Top 0.203: TP20.TESTPOINT J7.P0.19 53.98,72.64 49.53,77.09 40.01,77.09 35.81,77.09 v34.92,76.2 34.92,72.39 | v60.71,105.16 59.69,104.14 U2.5 | v60.71,105.16 60.71,106.3 U4.3 | U5.6 56.37,105.14 v56.39,105.16 | U3.23 34.26,71.72 34.92,72.39 | J3.1 40.64,16.05 v40.64,58.42 | R11.1 55.35,97.69 | 55.35,97.69 52.53,94.87 37.08,94.87 34.92,92.71 v34.92,81.28 | v60.71,105.16 62.23,103.63 62.23,99.69 60.33,97.79 55.45,97.79 55.35,97.69 | 34.92,72.39 39.37,72.39 40.64,71.12 v40.64,64.77
  Bottom 0.203: v56.39,105.16 v60.71,105.16 | v40.64,58.42 v40.64,64.77 | v34.92,81.28 v34.92,76.2
SENSORS_SDA  (via drill 0.2)
  Top 0.203: TP21.TESTPOINT J7.P0.20 51.44,79.63 34.54,79.63 33.66,78.74 | 58.67,106.17 58.67,106.3 U4.2 | U5.1 53.56,106.17 58.67,106.17 | 58.67,106.17 58.67,104.14 59.04,103.77 U2.6 57.82,103.16 53.77,99.11 R12.1 53.77,97.84 53.34,97.41 36.45,97.41 33.66,94.61 33.66,78.74 | U3.24 33.66,72.52 v33.66,73.66 33.66,78.74 | J3.2 41.91,16.78 v41.91,58.42 | v36.2,73.66 40.64,73.66 41.91,72.39 v41.91,64.77
  Bottom 0.203: v41.91,58.42 v41.91,64.77 | v36.2,73.66 v33.66,73.66
SWITCH_0  (via drill 0.2)
  Top 0.203: TP27.TESTPOINT J7.P0.22 | S4.IN 11.43,20.32 v11.43,22.23 | v16.51,22.23 19.05,24.77 19.05,38.73 v17.78,40.01 | v22.23,67.94 22.23,83.18 23.62,84.58 v30.48,84.58
  Bottom 0.203: v11.43,22.23 v16.51,22.23 | v17.78,40.01 17.78,63.5 v22.23,67.94 | J7.P0.22 49.02,84.58 37.34,84.58 v30.48,84.58
UART_RX
  Top 0.203: TP22.TESTPOINT J7.P0.08 49.53,34.29 49.53,21.86 54.61,16.78 J4.2 48.39,8.02 J1.1
UART_TX
  Top 0.203: TP23.TESTPOINT J7.P0.06 50.93,30.61 50.93,22.73 52.2,21.46 56.01,21.46 57.78,19.69 57.78,15.41 55.79,13.42 | J4.1 55.79,13.42 | 55.79,13.42 51.44,9.06 51.44,6.98 50.16,5.71 47.02,5.71 J1.2

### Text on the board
tPlace: RESET | TEMP & / HUMIDITY | POWER | PRESSURE | LIGHT | !LIGHT_INT | SD_EN | GROVE_D0 | SD Card | !LED_0 | !LED_1 | !LED_2 | I2C ACCELEROMETER / GYRO & MAGNETOMETER | SWITCH_0 | +Y | SDA | +Z | . | SCL | !LCD_CS | +X | LCD_SCLK | GND | LCD_MISO | GROVE_A1 | LCD_MOSI | GROVE_A0 | ANALOG / ACCELEROMETER | !SD_CS | !BUTTON_0 | ACCEL_X | SD_SCLK | +Y | SD_MISO | ACCEL_Y | +Z | . | ACCEL_Z | SD_MOSI | ACCEL / SELF TEST | +X | GND | GND | 0 | 1 | 2 | !IMU_INT | GROVE_D1 | Berkeley Buckler | Branden Ghena | B | BUTTON_0 | August 2018 | GND | GND | GND | GND | 3V3 | 3V3 | 3V3 | 3V3 | A1 | D1 | SDA | RX | A0 | D0 | SCL | TX | SWITCH_0 | GND | GND

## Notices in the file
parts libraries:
SparkFun-Aesthetics: Licensing: Creative Commons ShareAlike 4.0 International - https://creativecommons.org/licenses/by-sa/4.0
